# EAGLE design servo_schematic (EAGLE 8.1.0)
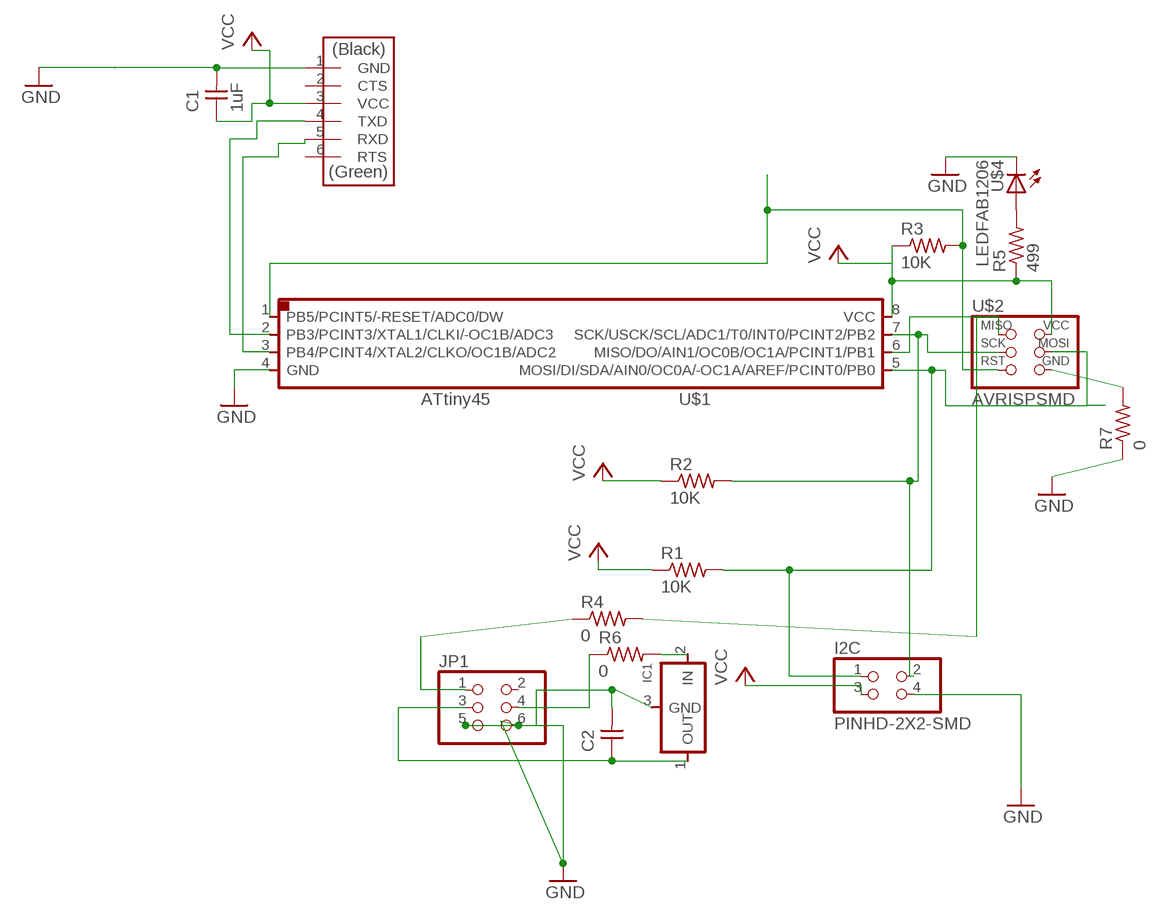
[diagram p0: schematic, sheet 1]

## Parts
C1  1uF  CAP-UNPOLARIZEDFAB  [C1206FAB]
C2  CAP-UNPOLARIZEDFAB  [C1206FAB]
I2C  PINHD-2X2-SMD  [2X02SMD]
IC1  REGULATORSOT23  [SOT23]
JP1  PINHD-2X3-SMD  [2X03SMD]
R1  10K  RES-US1206FAB  [R1206FAB]
R2  10K  RES-US1206FAB  [R1206FAB]
R3  10K  RES-US1206FAB  [R1206FAB]
R4  0  RES-US1206FAB  [R1206FAB]
R5  499  RES-US1206FAB  [R1206FAB]
R6  0  RES-US1206FAB  [R1206FAB]
R7  0  RES-US1206FAB  [R1206FAB]
U$1  ATTINY45SI  [SOIC8]
U$2  AVRISPSMD  [2X03SMD]
U$3  FTDI-SMD-HEADER  [1X06SMD]
U$4  LEDFAB1206  [LED1206FAB]

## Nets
GND: C1.2 C2.2 I2C.4 IC1.3(GND) JP1.5 JP1.6 R7.1 R7.2 U$1.4(GND) U$2.6(GND) U$3.1(GND) U$4.2(C)
N$1: I2C.2 R2.2 U$1.7(SCK/USCK/SCL/ADC1/T0/INT0/PCINT2/PB2) U$2.3(SCK)
N$2: R4.2 U$1.6(MISO/DO/AIN1/OC0B/OC1A/PCINT1/PB1) U$2.1(MISO)
N$3: I2C.1 R1.2 U$1.5(MOSI/DI/SDA/AIN0/OC0A/-OC1A/AREF/PCINT0/PB0) U$2.4(MOSI)
N$4: U$1.3(PB4/PCINT4/XTAL2/CLKO/OC1B/ADC2) U$3.5(RXD)
N$5: R3.2 U$1.1(PB5/PCINT5/-RESET/ADC0/DW) U$2.5(RST)
N$6: R5.2 U$4.1(A)
N$7: JP1.1 R4.1
N$8: C2.1 IC1.1(OUT) JP1.3
N$9: U$1.2(PB3/PCINT3/XTAL1/CLKI/-OC1B/ADC3) U$3.4(TXD)
N$10: IC1.2(IN) R6.2
N$12: JP1.4 R6.1
VCC: C1.1 I2C.3 R1.1 R2.1 R3.1 R5.1 U$1.8(VCC) U$2.2(VCC) U$3.3(VCC)
Unconnected: JP1.2 U$3.2(CTS) U$3.6(RTS)

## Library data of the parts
C1 C2 = fab:CAP-UNPOLARIZED
I2C = fab:PINHD-2X2-SMD
IC1 = fab:REGULATOR
JP1 = fab:PINHD-2X3-SMD: PIN HEADER
R1 R2 R4-R7 = fab:RES-US: Resistor (US Symbol)
R3 = fab:RES-US: Resistor (US Symbol); R1: 10K
U$1 = fab:ATTINY45
U$2 = fab:AVRISP
U$3 = fab:FTDI-SMD-HEADER
U$4 = fab:LED: LED

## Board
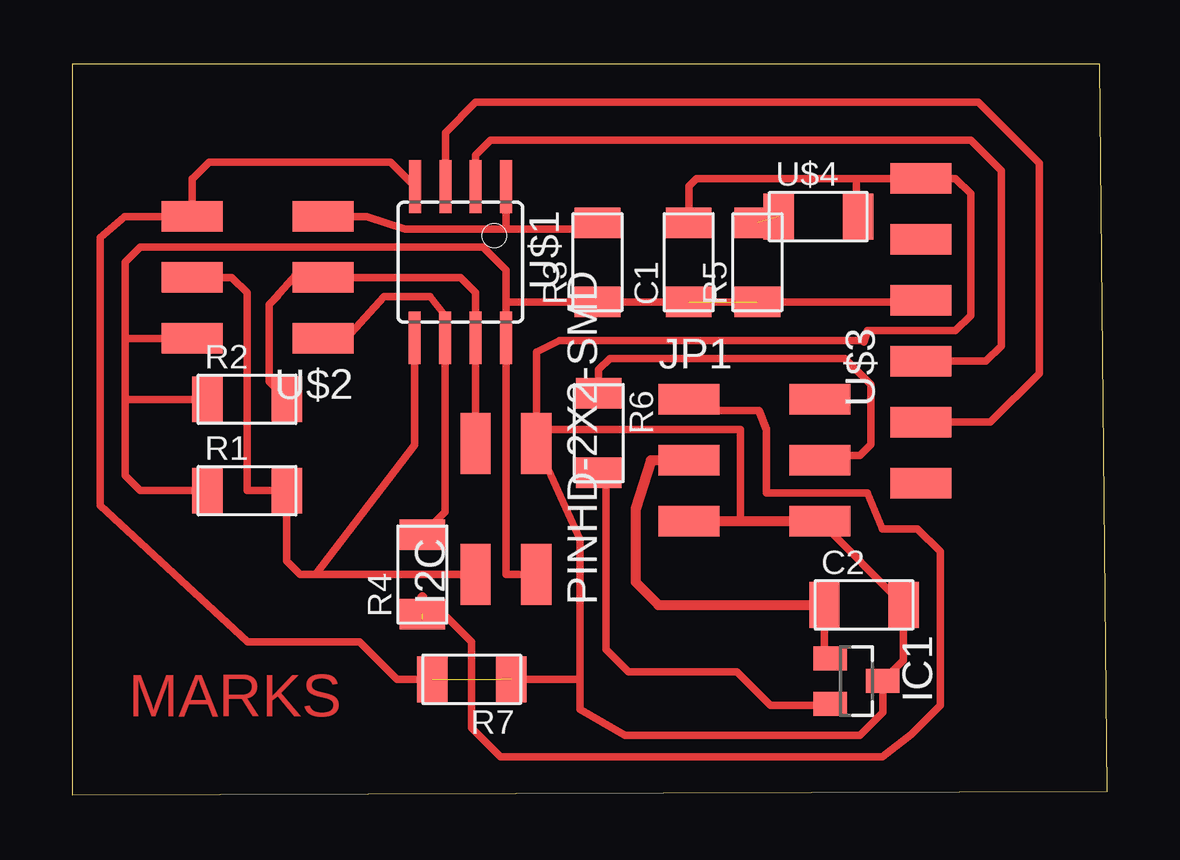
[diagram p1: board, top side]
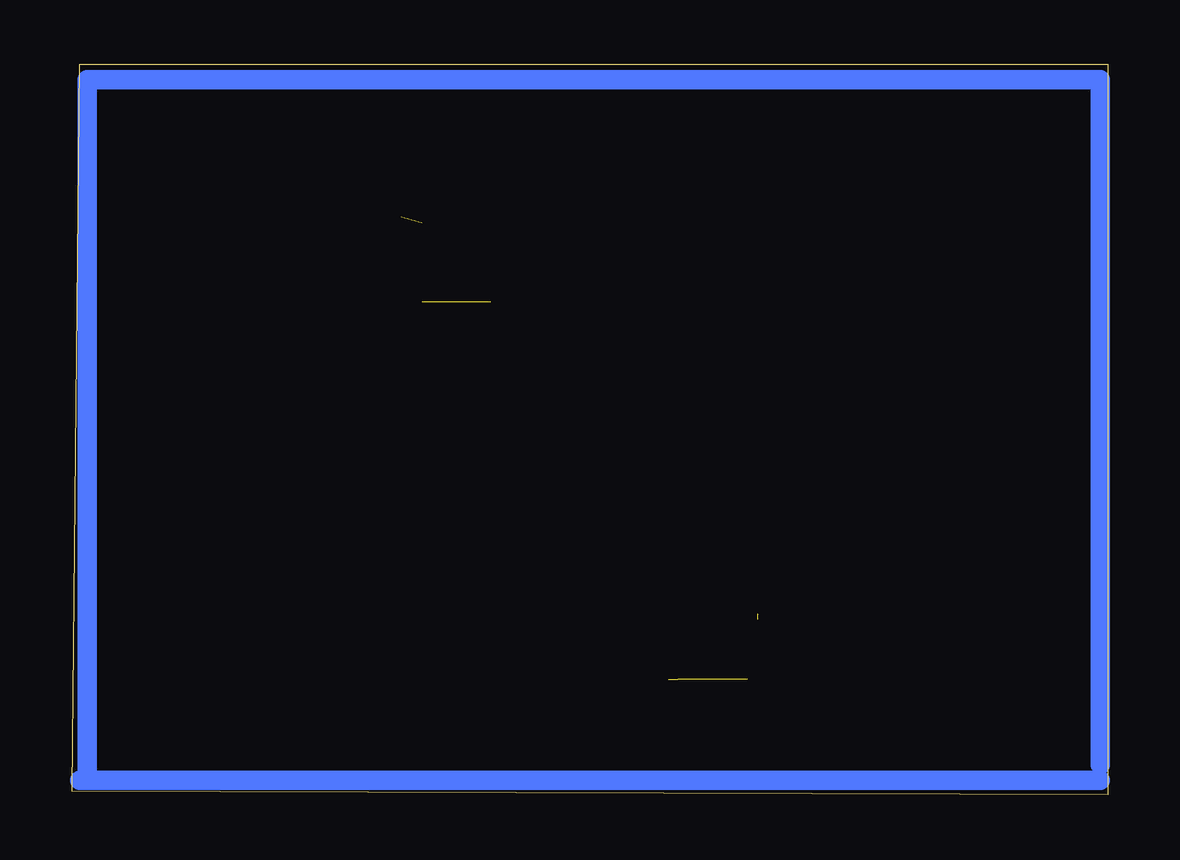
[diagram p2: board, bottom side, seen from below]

Size 43.16 x 30.47 mm. Coordinates in mm from the lower left corner, seen from the top.
Outline: 0,0 43.16,0.16 42.84,30.47 0,30.47 0,0
Copper layers (1*16): Top 0.035mm / dielectric 1.5mm / Bottom 0.035mm
Design rules "default": minimum track width 10mil, minimum drill 24mil, track to track 8mil, track to pad 8mil, pad to pad 8mil, via to via 8mil, smd to smd 8mil, copper to edge 40mil, drill to drill 8mil, minimum pad ring 10mil, minimum via ring 8mil, stop-mask expansion 4mil, vias tented up to drill 0mil, thermal gap 10mil

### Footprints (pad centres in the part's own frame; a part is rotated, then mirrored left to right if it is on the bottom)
C1206FAB = smd 1.27 x 1.905: 1 -1.651,0; 2 1.651,0
2X02SMD = smd 2.54 x 1.27: 1 -2.54,1.27; 2 2.92,1.27; 3 -2.54,-1.27; 4 2.92,-1.27
SOT23 = smd 1 x 1.4: 1 -0.95,-1.1; 2 0.95,-1.1; 3 0,1.1
2X03SMD = smd 2.54 x 1.27: 1 -2.54,2.54; 2 2.92,2.54; 3 -2.54,0; 4 2.92,0; 5 -2.54,-2.54; 6 2.92,-2.54
R1206FAB = smd 1.27 x 1.905: 1 -1.651,0; 2 1.651,0
SOIC8 = smd 0.5 x 2.2: 1 -1.905,-3.154; 2 -0.645,-3.154; 3 0.625,-3.154; 4 1.895,-3.154; 5 1.905,3.154; 6 0.635,3.154; 7 -0.635,3.154; 8 -1.905,3.154
1X06SMD = smd 2.54 x 1.27: 1 0,6.35; 2 0,3.81; 3 0,1.27; 4 0,-1.27; 5 0,-3.81; 6 0,-6.35
LED1206FAB = smd 1.27 x 1.905: 1 -1.651,0; 2 1.651,0

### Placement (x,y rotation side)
C1  25.71,22.21 90 top
C2  33.01,7.92 0 top
I2C  18.09,11.73 90 top
IC1  32.7,4.75 270 top
JP1  28.25,13.96 0 top
R1  7.3,12.69 0 top
R2  7.3,16.5 0 top
R3  21.9,22.21 90 top
R4  14.6,9.19 90 top
R5  28.57,22.21 90 top
R6  21.95,15.09 270 top
R7  16.66,4.82 180 top
U$1  16.19,22.21 180 top
U$2  7.93,21.58 180 top
U$3  35.39,19.35 0 top
U$4  31.11,24.12 0 top

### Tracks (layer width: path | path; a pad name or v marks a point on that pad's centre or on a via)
GND  (3 unrouted)
  Top 0.305: U$1.4 13.28,26.38 5.71,26.38 5.04,25.71 | 32.7,25.7 26.03,25.7 25.71,25.39 C1.2 | 32.7,25.7 U$3.1 36.82,25.7 37.46,25.07 37.46,19.99 36.82,19.36 33.16,19.36 33,18.89 33,18.95 20.32,18.95 19.36,18.46 19.36,15.25 | U$4.2 32.7,24.12 32.7,25.7 | 5.04,25.71 | 33.97,4.75 IC1.3 | 34.6,7.93 C2.2 | JP1.6 C2.2 | C2.2 34.67,5.62 IC1.3 | IC1.3 33.8,3.44 32.84,2.49 23.04,2.49 21.17,3.58 21.17,4.82 | 21.17,4.82 21.17,10.66 I2C.4 19.36,15.25 | 27.86,11.42 27.86,15.25 19.36,15.25 | 21.17,4.82 17.91,4.82 | 15.32,4.82 13.55,4.82 12,6.38 7.33,6.38 1.17,12.07 1.17,23.24 2.2,24.12 U$2.6 5.01,25.71 5.04,25.71
  Top 0.406: JP1.5 27.86,11.42 JP1.6
N$1
  Top 0.305: 8.32,20.56 8.21,20.45 8.21,17.23 R2.2 | 8.32,20.56 8.57,20.81 | I2C.2 U$1.7 16.82,20.94 16.19,21.58 U$2.3 9.52,21.9 8.32,20.56
N$2
  Top 0.305: R4.2 15.55,11.8 U$1.6 15.55,19.99 14.92,20.78 13.01,20.78 11.42,19.04 U$2.1
N$3
  Top 0.305: U$2.4 6.66,21.58 7.3,20.94 7.3,12.69 R1.2 8.95,9.77 9.52,9.19 10.15,9.19 | 10.15,9.19 I2C.1 | U$1.5 14.28,14.59 10.15,9.19
N$4
  Top 0.305: U$1.3 15.56,27.62 16.82,28.88 37.78,28.88 40.32,26.34 40.32,17.58 38.28,15.54 U$3.5
N$5
  Top 0.305: 21.85,23.91 R3.2 21.63,23.59 18.09,23.59 | 18.09,23.59 17.77,23.59 13.89,23.59 12.28,24.12 U$2.5 | U$1.1 18.09,23.59
N$6  (1 unrouted)
N$7  (1 unrouted)
  Top 0.305: 18.76,1.59 19,1.59 | 19,1.59 33.78,1.59 34.98,2.53 36.19,3.73 36.19,10.15 35.24,11.1 33.78,11.1 33.15,12.6 29.42,12.6 28.95,12.6 28.95,15.25 28.64,16.02 26.18,16.02 JP1.1 | R4.1 15.5,7.54 16.66,6.38 16.66,2.8 17.87,1.59 19,1.59
  Top 0.406: 14.6,7.31 14.6,8.24
N$8
  Top 0.305: IC1.1 31.36,5.7 C2.1
  Top 0.406: JP1.3 24.12,13.96 23.49,11.92 23.49,8.88 24.44,7.93 C2.1
N$9
  Top 0.305: U$3.4 38.09,18.08 38.73,18.72 38.73,26.02 37.46,27.29 17.46,27.29 16.83,26.67 U$1.2
N$10
  Top 0.305: R6.2 22.26,13.91 22.26,6.07 23.2,5.13 27.71,5.13 29.11,3.73 31.53,3.73 IC1.2
N$11
  Bottom 0.813: 0.31,0.62 42.54,0.62 | 42.86,0.62 42.54,0.62 | 42.54,0.62 42.54,29.83 0.31,29.83 0.31,1.26
N$12
  Top 0.305: JP1.4 31.17,14.16 32.84,14.16 33.31,14.62 33.31,17.11 32.22,18.2 22.42,18.2 21.95,17.74 R6.1
VCC  (1 unrouted)
  Top 0.305: 18.09,20.56 U$1.8 18.09,9.19 I2C.3 | 18.09,20.56 18.09,21.9 17.14,22.85 2.85,22.85 2.22,22.21 2.22,19.04 | 2.22,16.5 R2.1 | 2.22,19.04 2.22,16.5 | R1.1 2.85,12.69 2.22,13.32 2.22,16.5 | 18.09,20.56 R3.1 C1.1 34.92,20.56 U$3.3 | U$2.2 2.22,19.04

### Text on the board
Top: MARKS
